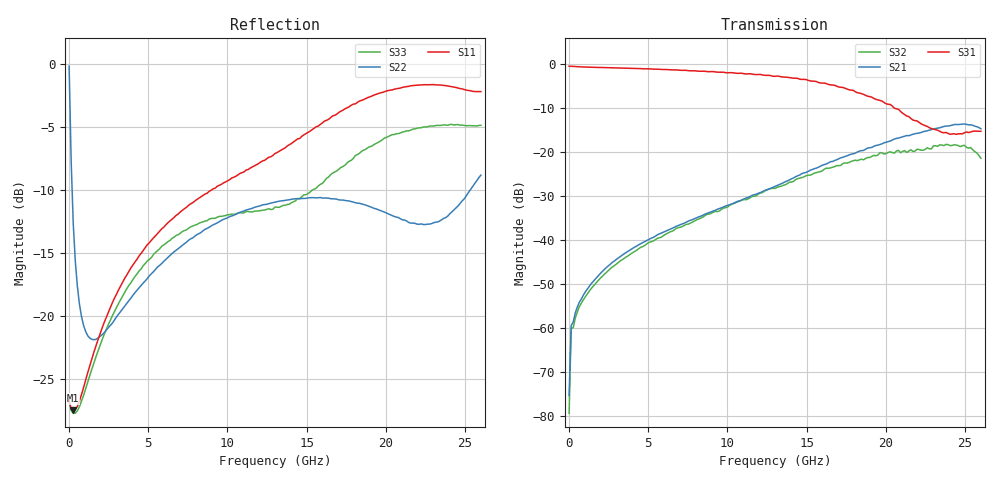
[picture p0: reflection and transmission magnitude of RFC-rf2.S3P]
!  3-Port S-parameters saved by WinCal
! VAR MeasName=S-Parameters (CALIBRATED_DATA) read from VNA (N5245A)
! VAR MeasDate=2016-7-4 10:45:26
! VAR NAME=25_C168105_RF2_RF3_10
! VAR FILENAME=25_C168105_RF2_RF3_10.S3P
! VAR DATE=2016-7-4 10:45:26
! VAR PHYS_PORTS=1,2,3
# Hz S DB R 50
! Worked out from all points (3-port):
!   201 points, 10 MHz to 26 GHz, reference 50 ohm
!   strongest paths, dB at 10 MHz, 6.508 GHz, 13.01 GHz, 19.5 GHz, 26 GHz:
!     S31: -0.6, -1.4, -2.9, -8.2, -15.3
!     S21: -75.3, -37.4, -27.8, -18.5, -14.8
!     S32: -79.3, -38.0, -28.3, -20.7, -21.5
!   lowest |S11| = -27.5 dB at 269.9 MHz (marker M1), VSWR 1.09, Z = 53.7 - j2.35 ohm
!   |S11| at or under -10 dB: start of sweep to 9.006 GHz
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1e7  -26.66 -5.4  -82.64 5.6  -0.57 -0.3
     -75.30 21.9  -0.19 -9.2  -78.52 45.0
     -0.58 -0.3  -79.29 47.0  -26.78 -5.1
1.3995e8  -27.36 -18.1  -59.16 46.5  -0.61 -2.1
          -59.42 46.4  -7.75 -65.6  -60.37 46.3
          -0.61 -2.1  -60.10 46.4  -27.51 -16.5
2.699e8  -27.47 -31.0  -58.66 38.8  -0.65 -3.8
         -58.59 40.2  -12.66 -77.2  -59.45 39.7
         -0.64 -3.8  -59.88 37.4  -27.71 -28.5
6.5975e8  -26.75 -59.1  -54.14 51.5  -0.73 -8.4
          -54.06 51.8  -19.04 -86.4  -55.01 50.1
          -0.73 -8.5  -55.06 50.3  -27.20 -54.4
1.43945e9  -23.40 -87.6  -49.82 59.0  -0.83 -17.4
           -49.76 58.7  -21.84 -93.2  -50.80 55.0
           -0.82 -17.4  -50.85 55.4  -24.22 -81.9
6.7674e9  -12.02 -166.0  -36.96 49.4  -1.45 -78.9
          -36.89 49.7  -14.78 -130.4  -37.37 32.3
          -1.43 -78.6  -37.36 32.7  -13.61 -158.8
1.3005e10  -7.11 138.3  -28.05 18.3  -2.96 -152.2
           -27.85 17.3  -10.97 179.6  -28.33 -28.1
           -2.88 -152.8  -28.31 -27.5  -11.36 92.7
1.807305e10  -3.18 95.9  -20.58 -34.5  -6.94 138.7
             -20.30 -32.9  -11.01 126.6  -22.26 -94.5
             -6.37 139.4  -21.90 -94.8  -7.28 -31.5
2.13218e10  -1.81 64.3  -16.35 -74.6  -11.88 111.9
            -16.31 -78.6  -12.47 86.9  -20.00 -146.1
            -11.88 105.9  -20.15 -147.4  -5.31 -89.4
2.6e10  -2.21 27.9  -14.83 -173.9  -15.24 104.8
        -14.78 -176.8  -8.83 30.9  -21.34 110.3
        -15.34 100.9  -21.46 110.3  -4.88 -139.3
